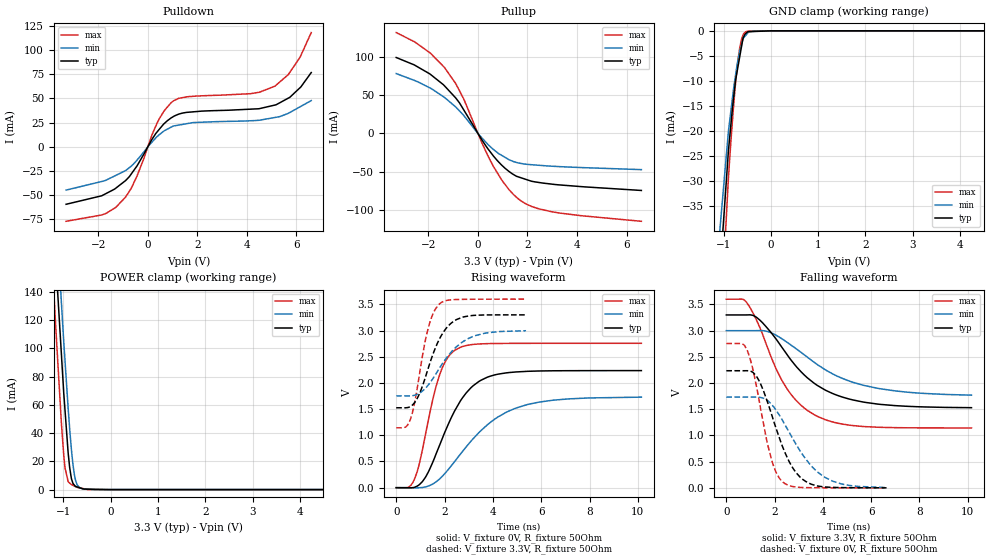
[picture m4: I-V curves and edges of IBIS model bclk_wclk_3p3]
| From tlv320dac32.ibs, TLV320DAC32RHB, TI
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|   bclk_wclk_3p3 Model
[Model]   bclk_wclk_3p3
Model_type   I/O
Polarity   Non-Inverting
Enable   Active-Low
Vinl = 0.99
Vinh = 2.31
Vmeas = 1.65
Vref = 1.65
Cref = 10pF
Rref = 50
|   typ   min   max
|   (nom PVT)   (fast PVT)   (slow PVT)
|C_comp from frequency sweep method (F=14MHz)
|Average
|C_comp   3.064e-12   2.812e-12   3.271e-12
|ON state : BUFFER OUTPUT TURNED HIGH
|C_comp   4.318e-12   3.830e-12   4.719e-12
|OFF state: BUFFER IN HIGH IMPEDANCE
|C_comp   1.810e-12   1.793e-12   1.822e-12
|C_comp from LC tank measurement(L=1nH)
|Average
|Resonant Frequency(Hz)   4.395e+09   4.420e+09   4.335e+09
|C_comp   1.322e-12   1.306e-12   1.363e-12
|ON state : BUFFER OUTPUT TURNED HIGH
|Resonant Frequency(Hz)   4.180e+09   4.220e+09   4.080e+09
|C_comp   1.451e-12   1.424e-12   1.523e-12
|OFF state: BUFFER IN HIGH IMPEDANCE
|Resonant Frequency(Hz)   4.610e+09   4.620e+09   4.590e+09
C_comp   1.193e-12   1.188e-12   1.204e-12
[Model spec]
|subparameter   typ   min   max
Vinl   0.99   0.90   1.08
Vinh   2.31   2.1   2.52
| Where nom  PVT is Nominal Process, 3.3V, 45C
|   Fast PVT is Strong Process,  3.6V, -40C
|   Slow PVT is Weak Process,   3V, 105C
[Voltage Range]   3.3   3   3.6
|Ambient Temperature   25   85   -40
|Junction Temperature
[Temperature Range]   45   105   -40
[Pullup Reference]   3.3   3   3.6
[Pulldown Reference]   0   0   0
[Power Clamp Reference]   3.3   3   3.6
[GND Clamp Reference]   0   0   0
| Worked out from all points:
|   slope of the pulldown table from 0 to 0.495 V, typ, clamps not added: 25.9 ohm
|   slope of the pullup table from 0 to 0.495 V, typ, clamps not added: 20.6 ohm
|   GND clamp passes 1 mA (typ) near -0.56 V on its own axis
|   POWER clamp passes 1 mA (typ) near -0.63 V on its own axis
|   falling waveform, V_fixture 3.3V, R_fixture 50Ohm: 20-80 % time 2.15ns typ, 2.65ns min, 1.62ns max; typ from 3.3 V to 1.53 V
|   rising waveform, V_fixture 0V, R_fixture 50Ohm: 20-80 % time 1.39ns typ, 2.18ns min, 834ps max; typ from 0 V to 2.23 V
|   rising waveform, V_fixture 3.3V, R_fixture 50Ohm: 20-80 % time 882ps typ, 1.25ns min, 595ps max; typ from 1.52 V to 3.3 V
|   falling waveform, V_fixture 0V, R_fixture 50Ohm: 20-80 % time 1.08ns typ, 1.47ns min, 741ps max; typ from 2.23 V to 0.001 V
[Pulldown]
|   Voltage   I(typ)   I(min)   I(max)
-3.3V     -59.42mA   -44.74mA   -77.02mA
-1.696V   -48.42mA   -34.59mA   -68.97mA
-896.4mV  -34.87mA   -24.56mA   -51.93mA
-435.6mV  -19.73mA   -13.76mA   -30.16mA
381.6mV   15.62mA    10.8mA     24.88mA
1.008V    30.93mA    21.24mA    47.01mA
1.591V    35.68mA    24.02mA    51.77mA
4.162V    38.99mA    26.97mA    54.99mA
5.134V    43.21mA    30.37mA    62.79mA
5.67V     50.3mA     34.59mA    74.6mA
6.149V    61.17mA    41.41mA    92.66mA
6.6V      76.84mA    47.84mA    118.2mA
[GND Clamp]
|   Voltage   I(typ)   I(min)   I(max)
-3.3V     -1.363A    -1.215A    -1.557A
-1.501V   -106.7mA   -86.11mA   -137.1mA
-897.6mV  -24.09mA   -20.19mA   -29.58mA
-792mV    -13.73mA   -11.9mA    -15.51mA
-745.8mV  -9.895mA   -8.859mA   -10.43mA
-702mV    -7.547mA   -6.224mA   -6.431mA
-622.8mV  -3.301mA   -2.892mA   -1.787mA
-590.7mV  -1.58mA    -1.753mA   -927.4uA
-532.8mV  -561.8uA   -927.8uA   -190.4uA
-465mV    -178.6uA   -178uA     -58.72uA
-285mV    -109uA     -2.294uA   -4.272uA
6.6V      0A         0A         0A
[Pullup]
|   Voltage   I(typ)   I(min)   I(max)
-3.3V     99.36mA    78.34mA    132mA
-1.94V    77.87mA    59.58mA    105.6mA
-1.35V    62.26mA    47.16mA    86.22mA
-896.4mV  46.41mA    34.64mA    65.25mA
-579.6mV  31.15mA    23.81mA    45.5mA
172.8mV   -9.103mA   -6.287mA   -13.21mA
633.6mV   -29.89mA   -21.27mA   -43.6mA
1.246V    -49.58mA   -34.22mA   -73.23mA
1.706V    -57.71mA   -39.1mA    -87.56mA
2.167V    -62.64mA   -40.97mA   -95.57mA
3.087V    -66.78mA   -43.1mA    -103.1mA
6.6V      -74.66mA   -47.41mA   -115mA
[POWER Clamp]
|   Voltage   I(typ)   I(min)   I(max)
-3.3V     1.555A     1.564A     1.556A
-1.361V   288.8mA    321.6mA    241.4mA
-1.166V   168.8mA    205mA      119.1mA
-1.119V   139.5mA    176.9mA    91.96mA
-1.04V    96.13mA    132.8mA    47.35mA
-964.8mV  56.73mA    91.82mA    15.61mA
-897.6mV  26.14mA    57.67mA    5.749mA
-831.6mV  8.397mA    29.7mA     3.661mA
-768mV    3.259mA    11.1mA     2.56mA
-705.6mV  1.885mA    3.349mA    1.586mA
-336mV    214.7uA    7.125uA    7.046uA
6.6V      0A         0A         0A
[Ramp]
R_load = 50
|   typ   min   max
dV/dt_r   1.34124/1.38397e-09   1.03901/2.18537e-09   1.65397/8.32037e-10
dV/dt_f   1.06461/2.15556e-09   0.747718/2.72806e-09   1.47416/1.62092e-09
[Falling Waveform]
V_fixture = 3.3V
V_fixture_min = 3V
V_fixture_max = 3.6V
R_fixture = 50Ohm
|   Time   V(typ)   V(min)   V(max)
0s        3.3V       3V         3.6V
836ps     3.3V       3V         3.543V
1.372ns   3.209V     3.002V     3.078V
1.888ns   2.944V     2.954V     2.461V
2.328ns   2.666V     2.837V     2.031V
2.928ns   2.3V       2.643V     1.652V
3.744ns   1.963V     2.362V     1.372V
4.812ns   1.732V     2.089V     1.217V
6.268ns   1.599V     1.9V       1.157V
10.16ns   1.53V      1.769V     1.144V
[Rising Waveform]
V_fixture = 0V
V_fixture_min = 0V
V_fixture_max = 0V
R_fixture = 50Ohm
|   Time   V(typ)   V(min)   V(max)
0s        2.496nV    20.4nV     793.1pV
496ps     -2.164mV   43.41uV    5.859mV
760ps     7.962mV    -2.058mV   167.4mV
1.224ns   209.5mV    16.05mV    1.047V
1.768ns   778.9mV    155.6mV    2.116V
2.08ns    1.132V     306.2mV    2.448V
2.416ns   1.464V     498.7mV    2.621V
3.424ns   2.028V     1.052V     2.744V
4.952ns   2.209V     1.519V     2.755V
10.14ns   2.235V     1.728V     2.757V
[Rising Waveform]
V_fixture = 3.3V
V_fixture_min = 3V
V_fixture_max = 3.6V
R_fixture = 50Ohm
|   Time   V(typ)   V(min)   V(max)
0s        1.525V     1.753V     1.143V
384ps     1.525V     1.753V     1.156V
588ps     1.55V      1.753V     1.306V
924ps     1.754V     1.795V     2.051V
1.256ns   2.18V      1.921V     2.917V
1.508ns   2.532V     2.075V     3.305V
1.788ns   2.838V     2.28V      3.508V
2.32ns    3.157V     2.611V     3.589V
3.168ns   3.288V     2.885V     3.598V
5.372ns   3.299V     2.996V     3.6V
[Falling Waveform]
V_fixture = 0V
V_fixture_min = 0V
V_fixture_max = 0V
R_fixture = 50Ohm
|   Time   V(typ)   V(min)   V(max)
0s        2.235V     1.732V     2.757V
656ps     2.235V     1.732V     2.754V
872ps     2.236V     1.732V     2.616V
1.092ns   2.206V     1.732V     2.277V
1.356ns   2.044V     1.729V     1.678V
1.892ns   1.379V     1.585V     510.5mV
2.348ns   765.2mV    1.272V     108mV
3.068ns   200.7mV    697.5mV    8.774mV
4.02ns    19.65mV    219.8mV    1.719mV
6.64ns    850.8uV    6.335mV    233.4uV
